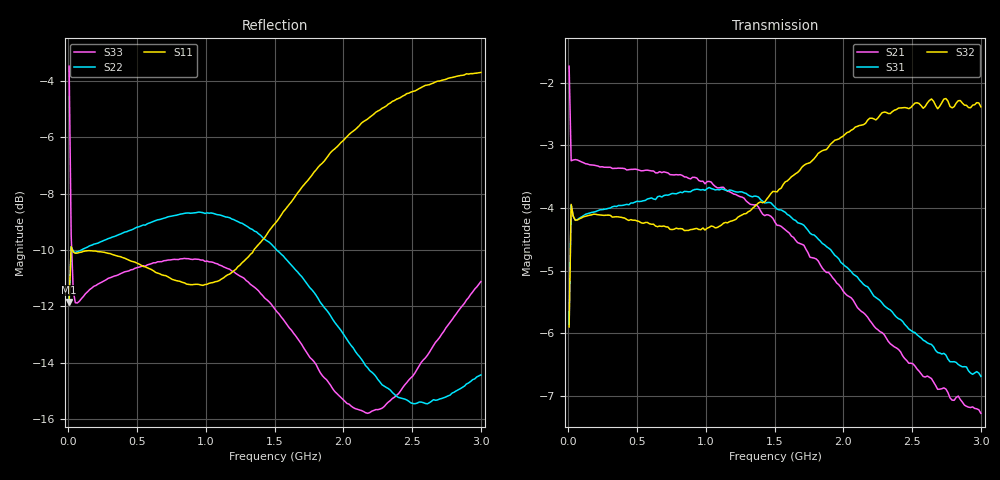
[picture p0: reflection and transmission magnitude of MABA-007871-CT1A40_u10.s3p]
#	MHz	S	RI	R	50
!FREQ	R1	I1	R2	I2	R3	I3
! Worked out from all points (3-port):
!   201 points, 5 MHz to 3 GHz, reference 50 ohm
!   strongest paths, dB at 5 MHz, 753.8 MHz, 1.502 GHz, 2.251 GHz, 3 GHz:
!     S32: -5.9, -4.3, -3.7, -2.6, -2.4
!     S31: -5.9, -3.8, -4.0, -5.5, -6.7
!     S21: -1.7, -3.5, -4.2, -5.9, -7.3
!   lowest |S11| = -11.8 dB at 5 MHz (marker M1), VSWR 1.69, Z = 70.3 + j23.9 ohm
!   |S11| at or under -10 dB: start of sweep to 19.08 MHz; 29.37 MHz to 1.349 GHz (1.32 GHz wide, 191 % of centre)
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5  0.2005 0.1588  0.8007 -0.1645  -0.4001 -0.315
   0.8022 -0.1652  0.1979 0.1609  0.3974 0.3169
   -0.4001 -0.315  0.3938 0.3192  -0.2049 0.6388
19.975  0.3175 0.0436  0.6846 -0.0683  -0.628 -0.0909
        0.6848 -0.0685  0.3161 0.0542  0.6266 0.1014
        -0.628 -0.0909  0.6271 0.1009  0.259 0.2128
64.9  0.3119 -0.0146  0.6861 -0.0661  -0.6175 0.0124
      0.686 -0.0661  0.3134 0.0185  0.6169 0.0209
      -0.6175 0.0124  0.6168 0.0209  0.2445 0.0712
843.6  -0.00696 -0.2764  0.3897 -0.5487  -0.3714 0.534
       0.391 -0.5417  0.3611 -0.0675  0.5968 -0.1116
       -0.3714 0.534  0.5945 -0.1135  0.3039 -0.032
1158.075  -0.2147 -0.1885  0.1459 -0.635  -0.1454 0.6348
          0.1569 -0.6316  0.3374 -0.1303  0.5995 -0.1371
          -0.1454 0.6348  0.5979 -0.1393  0.2835 -0.0743
1502.5  -0.3484 0.053  -0.1333 -0.5936  0.1189 0.6207
        -0.12 -0.6028  0.2675 -0.1734  0.627 -0.1833
        0.1189 0.6207  0.6234 -0.1851  0.229 -0.096
1816.975  -0.3114 0.3165  -0.3245 -0.4511  0.3053 0.5117
          -0.3215 -0.4735  0.1987 -0.1663  0.6527 -0.2589
          0.3053 0.5117  0.6486 -0.2571  0.1804 -0.0726
2236.275  -0.0561 0.553  -0.4376 -0.2051  0.4333 0.3141
          -0.4556 -0.2194  0.1507 -0.1133  0.6364 -0.4
          0.4333 0.3141  0.6282 -0.3948  0.1645 -0.00792
2595.675  0.2249 0.5779  -0.4413 -0.0147  0.4653 0.1651
          -0.4622 -0.0108  0.1532 -0.0709  0.5729 -0.5207
          0.4653 0.1651  0.5671 -0.507  0.1996 0.0386
3000  0.4808 0.443  -0.3845 0.1674  0.4625 0.0172
      -0.3903 0.1861  0.1815 -0.0553  0.4454 -0.6305
      0.4625 0.0172  0.4422 -0.618  0.2732 0.0514
